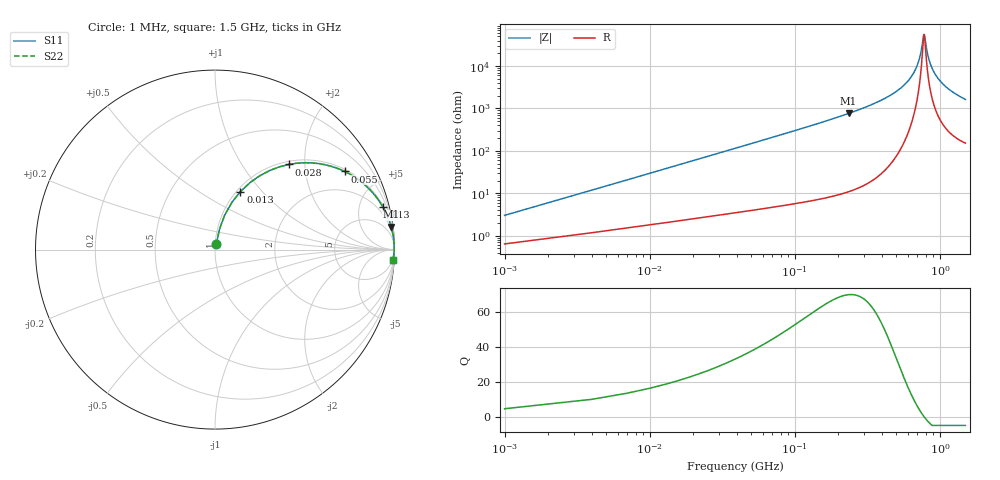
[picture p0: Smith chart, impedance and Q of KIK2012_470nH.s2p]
!version-2
!date-01.2022
!Series
# MHz S RI R 50
!Freq ReS11 ImS11 ReS21 ImS21 ReS12 ImS12 ReS22 ImS22
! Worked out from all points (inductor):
!   501 points, 1 MHz to 1.5 GHz, reference 50 ohm
!   read as one part in series: L = 470 nH near 7 MHz
!   highest Q = 70.2 at 235 MHz (marker M1), where L = 517 nH
!   self-resonance near 778 MHz
!   S11 on the Smith chart (normalised r, x): 1 MHz: 1.01, +0.06; 13 MHz: 1.04, +0.77; 28 MHz: 1.06, +1.66; 55 MHz: 1.08, +3.26; 130 MHz: 1.13, +7.90; 1.5 GHz: 4, -33
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1  0.00722 0.0291  0.9928 -0.0291  0.9928 -0.0291  0.00722 0.0291
10  0.094 0.2629  0.906 -0.2629  0.906 -0.2629  0.094 0.2629
13  0.1416 0.3231  0.8584 -0.3231  0.8584 -0.3231  0.1416 0.3231
19  0.2493 0.4114  0.7507 -0.4114  0.7507 -0.4114  0.2493 0.4114
28  0.4102 0.4744  0.5898 -0.4744  0.5898 -0.4744  0.4102 0.4744
55  0.7222 0.4354  0.2778 -0.4354  0.2778 -0.4354  0.7222 0.4354
85  0.8609 0.336  0.1391 -0.336  0.1391 -0.336  0.8609 0.336
130  0.9363 0.236  0.0637 -0.236  0.0637 -0.236  0.9363 0.236
235  0.9814 0.1283  0.0186 -0.1283  0.0186 -0.1283  0.9814 0.1283
253  0.9842 0.1176  0.0158 -0.1176  0.0158 -0.1176  0.9842 0.1176
502  0.9973 0.0393  0.00272 -0.0393  0.00272 -0.0393  0.9973 0.0393
667  0.9984 0.0135  0.00165 -0.0135  0.00165 -0.0135  0.9984 0.0135
715  0.9983 0.00743  0.00165 -0.00743  0.00165 -0.00743  0.9983 0.00743
751  0.9983 0.00317  0.00171 -0.00317  0.00171 -0.00317  0.9983 0.00317
772  0.9982 0.000779  0.00177 -0.000779  0.00177 -0.000779  0.9982 0.000779
781  0.9982 -0.000224  0.0018 0.000224  0.0018 0.000224  0.9982 -0.000224
823  0.998 -0.00476  0.00197 0.00476  0.00197 0.00476  0.998 -0.00476
862  0.9978 -0.00877  0.00217 0.00877  0.00217 0.00877  0.9978 -0.00877
922  0.9975 -0.0146  0.00255 0.0146  0.00255 0.0146  0.9975 -0.0146
1003  0.9968 -0.022  0.00318 0.022  0.00318 0.022  0.9968 -0.022
1252  0.9942 -0.0423  0.00582 0.0423  0.00582 0.0423  0.9942 -0.0423
1500  0.9907 -0.0599  0.0093 0.0599  0.0093 0.0599  0.9907 -0.0599
